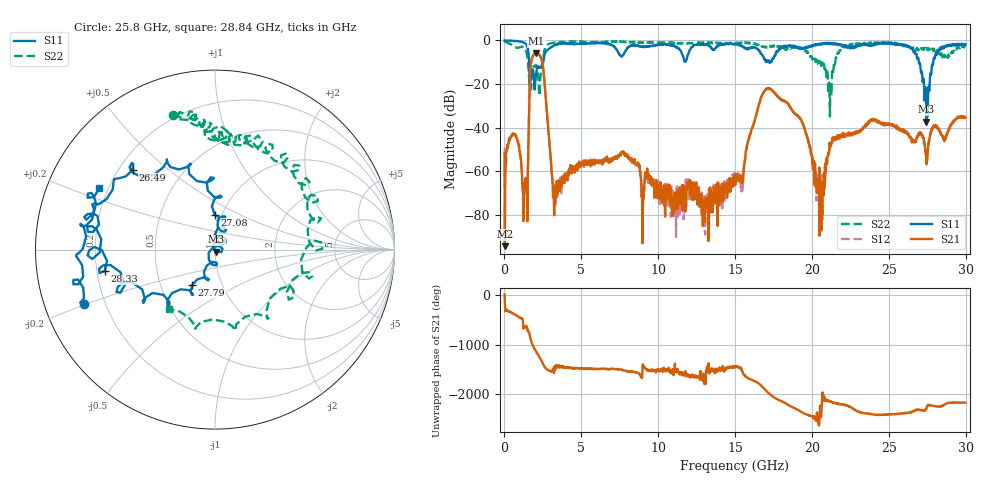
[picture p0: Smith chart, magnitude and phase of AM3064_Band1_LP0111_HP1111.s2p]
# Hz S DB R 50.0
!freq dBS11 angS11 dBS21 angS21 dBS12 angS12 dBS22 angS22
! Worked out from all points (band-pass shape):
!   1600 points, 10 MHz to 29.98 GHz, reference 50 ohm
!   highest |S21| = -5.95 dB at 2.072 GHz (marker M1); lowest = -94.4 dB at 28.74 MHz (marker M2)
!   |S21| within 3 dB of the highest: 1.762 GHz to 2.423 GHz (660.8 MHz wide, 31.6 % of centre)
!   lowest |S11| = -37.3 dB at 27.45 GHz (marker M3), VSWR 1.03, Z = 50.7 - j1.18 ohm
!   |S11| at or under -10 dB: 1.6 GHz to 2.522 GHz (922.5 MHz wide, 44.8 % of centre); 17.24139 GHz to 17.29264 GHz (51.25 MHz wide, 0.297 % of centre); 26.95 GHz to 27.89 GHz (939.3 MHz wide, 3.43 % of centre)
!   |S22| runs from -34.9 to -0.3 dB; largest |S21 - S12| = 0.0081
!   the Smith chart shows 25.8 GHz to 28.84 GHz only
!   S11 on the Smith chart (normalised r, x): 25.8 GHz: 0.12, -0.19; 26.49 GHz: 0.25, +0.38; 27.08 GHz: 0.92, +0.37; 27.79 GHz: 0.72, -0.30; 28.33 GHz: 0.23, -0.09; 28.84 GHz: 0.17, +0.24
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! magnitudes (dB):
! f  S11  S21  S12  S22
! 10 MHz  -0.1  -51.8  -49.3  -0.3
! 28.74 MHz  -0.1  -94.4  -67.6  -0.5
! 1.36 GHz  -1.5  -68.1  -70.3  -4.0
! 1.753 GHz  -14.8  -9.2  -9.2  -19.8
! 2.072 GHz  -14.8  -6.0  -5.9  -11.6
! 3.234 GHz  -2.3  -80.2  -69.2  -1.0
! 5.015 GHz  -1.4  -56.3  -56.9  -0.6
! 10 GHz  -2.1  -67.2  -70.7  -1.0
! 15 GHz  -1.8  -61.6  -63.1  -1.3
! 17.1 GHz  -9.4  -22.1  -22.1  -3.0
! 19.99 GHz  -2.9  -52.9  -53.5  -7.9
! 20.65 GHz  -1.5  -67.5  -67.2  -10.0
! 21.47 GHz  -1.5  -44.4  -44.3  -10.7
! 25 GHz  -1.1  -38.5  -38.2  -1.2
! 25.8 GHz  -2.0  -41.2  -41.5  -2.1
! 26.49 GHz  -3.9  -46.8  -45.6  -3.5
! 27.08 GHz  -14.3  -42.6  -42.4  -3.9
! 27.45 GHz  -37.3  -56.8  -56.7  -3.5
! 27.79 GHz  -12.6  -40.4  -41.0  -4.1
! 28.33 GHz  -4.1  -42.3  -42.0  -6.1
! 28.84 GHz  -2.7  -41.9  -41.8  -7.5
! 29.98 GHz  -1.8  -35.5  -35.5  -2.8
